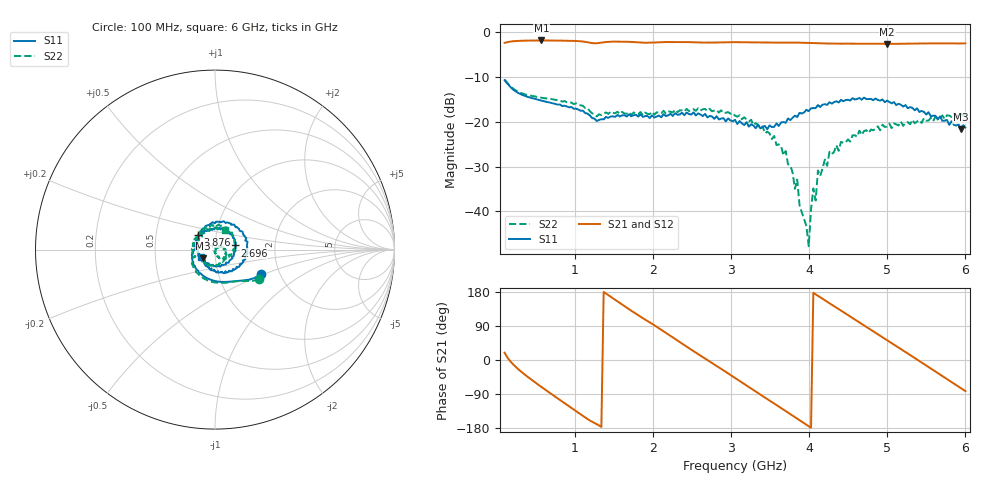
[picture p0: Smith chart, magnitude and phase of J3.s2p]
!Agilent Technologies,E8364B,MY43040379,A.07.50.67
!Agilent E8364B: A.07.50.67
!Date: Tuesday, March 24, 2026 11:05:46
!Correction: S11(Full 2 Port(1,2))
!S21(Full 2 Port(1,2))
!S12(Full 2 Port(1,2))
!S22(Full 2 Port(1,2))
!S2P File: Measurements: S11, S21, S12, S22:
# Hz S  dB  R 50
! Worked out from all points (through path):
!   201 points, 100 MHz to 6 GHz, reference 50 ohm
!   highest |S21| = -1.82 dB at 572 MHz (marker M1); lowest = -2.6 dB at 4.997 GHz (marker M2)
!   group delay of S21, straight-line fit = 375 ps
!   lowest |S11| = -21.7 dB at 5.941 GHz (marker M3), VSWR 1.18, Z = 43.7 - j4.35 ohm
!   |S11| at or under -10 dB: start of sweep to end of sweep
!   |S22| runs from -47.8 to -10.6 dB; largest |S21 - S12| = 0.0043
!   S11 on the Smith chart (normalised r, x): 100 MHz: 1.61, -0.48; 2.696 GHz: 1.24, +0.06; 3.876 GHz: 0.82, +0.14; 6 GHz: 0.86, -0.07
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1e8  -10.72 -27.9  -2.35 19.3  -2.36 19.0  -10.57 -34.0
3.065e8  -13.83 -60.6  -1.89 -29.8  -1.91 -30.0  -13.53 -57.1
5.72e8  -15.26 -93.5  -1.82 -71.3  -1.84 -71.5  -14.63 -84.2
1.103e9  -17.51 -166.8  -2.05 -147.5  -2.07 -147.8  -16.42 -148.7
1.5455e9  -18.46 153.9  -2.07 154.7  -2.08 154.5  -17.75 178.4
2.0765e9  -18.60 93.7  -2.23 83.7  -2.24 83.5  -18.03 131.6
2.696e9  -19.01 12.1  -2.30 -0.1  -2.33 -0.3  -17.59 67.6
3.05e9  -19.56 -44.6  -2.20 -47.4  -2.21 -47.7  -18.62 19.6
3.3745e9  -21.46 -115.8  -2.30 -91.3  -2.32 -91.5  -21.58 -19.1
3.699e9  -20.22 175.8  -2.29 -134.7  -2.30 -134.9  -26.53 -67.7
3.8465e9  -18.92 143.9  -2.30 -154.8  -2.32 -155.0  -32.90 -86.0
3.876e9  -18.02 138.7  -2.32 -158.9  -2.34 -159.1  -38.61 -111.8
3.994e9  -17.63 115.2  -2.36 -174.9  -2.38 -175.0  -47.79 8.9
4.053e9  -16.94 103.3  -2.39 177.2  -2.41 177.2  -34.88 32.6
4.0825e9  -16.95 102.7  -2.42 173.3  -2.43 173.0  -37.60 52.5
4.2595e9  -15.62 72.8  -2.51 149.9  -2.53 149.7  -26.71 20.9
4.584e9  -15.00 27.2  -2.54 107.0  -2.55 106.9  -23.00 -35.3
4.997e9  -15.26 -22.9  -2.59 52.2  -2.60 52.1  -21.05 -101.5
5.0265e9  -15.56 -30.0  -2.57 48.4  -2.59 48.4  -20.42 -112.1
5.469e9  -17.78 -81.8  -2.50 -10.5  -2.51 -10.6  -19.20 160.9
5.941e9  -21.71 -142.9  -2.49 -74.2  -2.50 -74.3  -18.07 70.1
6e9  -21.29 -150.9  -2.48 -82.1  -2.50 -82.1  -18.14 63.4
